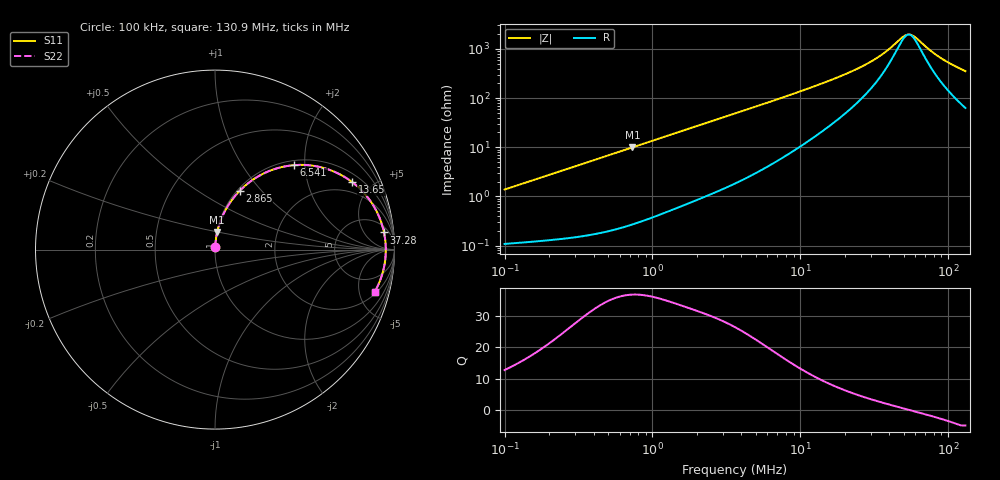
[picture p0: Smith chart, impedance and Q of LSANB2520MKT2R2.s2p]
! LSANB2520MKT2R2  S-PARAMETER MODEL  ( General Type )
! Model Generated by TAIYO YUDEN Corporation (http://www.ty-top.com)
! Version 1.0
! TAIYO YUDEN Control No. 120417NG38SB-FKC
! Copyright(c) 2012 TAIYO YUDEN CO.,LTD. All Rights Reserved.
! Product Description (link to TY-COMPAS)
! https://ds.yuden.co.jp/TYCOMPAS/or/detail?pn=LSANB2520MKT2R2M&u=M
! Products Name : Inductors
! Characteristics :
!  Inductance : 2.2 uH , SRF(min) : -Hz , DC Resistance(max) : 0.110 Ohm
!  Rated Current : Saturation :2000 mA , Temp Rise : 1900 mA (40 degC)
!  Case Size : 2.5 x 2.0 / 0.098 x 0.079 [mm/inch] , Thickness : 1.2 / 0.047 [mm/inch]
!  (Conditions: Temperature = 25 degC , DC Bias Current/Voltage = 0A / 0V)
! External Node Assignments :
!  1  o---GGG---o  2
! GND o---------o GND
! Frequency Range : 0.1MHz  -  130.914307MHz  [ 402 STEP ]
# MHz S RI R 50
! Freq[MHz].  S11 Real  S11 Imag  S21 Real  S21 Imag  S12 Real  S12 Imag  S22 Real  S22 Imag
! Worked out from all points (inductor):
!   401 points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, 100 kHz to 130.9 MHz, reference 50 ohm
!   read as one part in series: L = 2.19 uH near 103.7 kHz
!   highest Q = 36.9 at 732.8 kHz (marker M1), where L = 2.16 uH
!   self-resonance near 54.24 MHz
!   S11 on the Smith chart (normalised r, x): 100 kHz: 1.00, +0.03; 2.865 MHz: 1.03, +0.77; 6.541 MHz: 1.09, +1.76; 13.65 MHz: 1.39, +3.83; 37.28 MHz: 8, +15; 130.9 MHz: 2.26, -6.96
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0.1  0.00127 0.0138  0.9987 -0.0138  0.9987 -0.0138  0.00127 0.0138
0.332733  0.0036 0.0452  0.9964 -0.0452  0.9964 -0.0452  0.0036 0.0452
0.732764  0.0124 0.0981  0.9876 -0.0981  0.9876 -0.0981  0.0124 0.0981
1.10711  0.0259 0.1454  0.9741 -0.1454  0.9741 -0.1454  0.0259 0.1454
1.862826  0.0655 0.2324  0.9345 -0.2324  0.9345 -0.2324  0.0655 0.2324
2.865441  0.137 0.327  0.863 -0.327  0.863 -0.327  0.137 0.327
3.683715  0.2048 0.3849  0.7952 -0.3849  0.7952 -0.3849  0.2048 0.3849
6.541013  0.4405 0.4705  0.5595 -0.4705  0.5595 -0.4705  0.4405 0.4705
8.716146  0.5795 0.4612  0.4205 -0.4612  0.4205 -0.4612  0.5795 0.4612
12.03896  0.7199 0.406  0.2801 -0.406  0.2801 -0.406  0.7199 0.406
13.65011  0.7653 0.3754  0.2347 -0.3754  0.2347 -0.3754  0.7653 0.3754
24.67673  0.9031 0.2079  0.0969 -0.2079  0.0969 -0.2079  0.9031 0.2079
30.60534  0.9275 0.148  0.0725 -0.148  0.0725 -0.148  0.9275 0.148
37.2833  0.9417 0.0955  0.0583 -0.0955  0.0583 -0.0955  0.9417 0.0955
40.05754  0.9451 0.0769  0.0549 -0.0769  0.0549 -0.0769  0.9451 0.0769
50.58087  0.9513 0.0176  0.0487 -0.0176  0.0487 -0.0176  0.9513 0.0176
53.37817  0.9516 0.00402  0.0484 -0.00402  0.0484 -0.00402  0.9516 0.00402
56.33018  0.9516 -0.00953  0.0484 0.00953  0.0484 0.00953  0.9516 -0.00953
60.52168  0.9509 -0.0276  0.0491 0.0276  0.0491 0.0276  0.9509 -0.0276
75.06208  0.9446 -0.0827  0.0554 0.0827  0.0554 0.0827  0.9446 -0.0827
88.21711  0.9351 -0.1253  0.0649 0.1253  0.0649 0.1253  0.9351 -0.1253
130.9143  0.8896 -0.2358  0.1104 0.2358  0.1104 0.2358  0.8896 -0.2358
